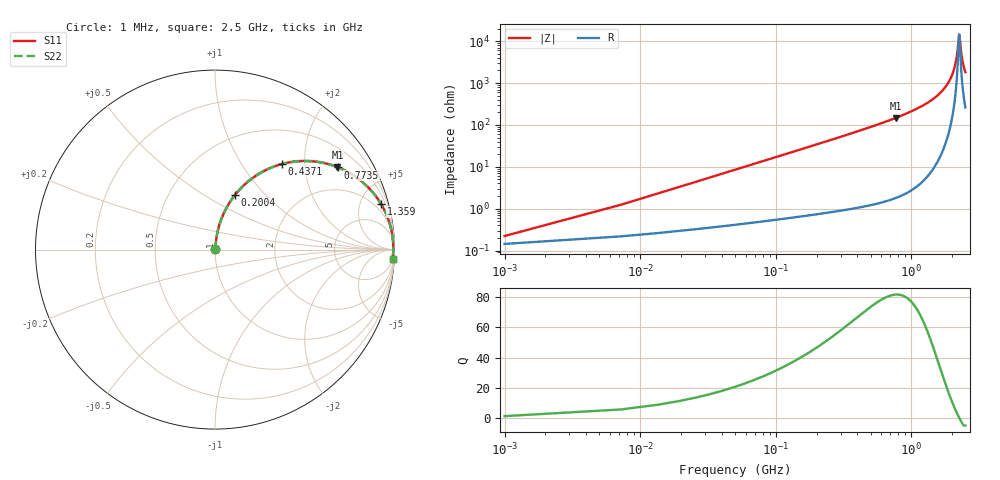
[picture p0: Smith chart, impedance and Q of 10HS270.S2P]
! Coilcraft 1008HS-270 Chip Inductor
! 02 July 2002
# MHZ S MA R 50
!Freq  MagS11  AngS11  MagS21  AngS21  MagS12  AngS12  MagS22  AngS22
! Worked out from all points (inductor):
!   403 points, 1 MHz to 2.5 GHz, reference 50 ohm
!   read as one part in series: L = 27 nH near 13.46 MHz
!   highest Q = 81.7 at 767.3 MHz (marker M1), where L = 30.5 nH
!   self-resonance near 2.25 GHz
!   S11 on the Smith chart (normalised r, x): 1 MHz: 1.00, +0.00; 200.4 MHz: 1.01, +0.69; 437.1 MHz: 1.02, +1.54; 773.5 MHz: 1.04, +2.98; 1.359 GHz: 1.13, +7.25; 2.5 GHz: 6, -36
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1  0.002223 49.6  0.9986 -0.1  0.9986 -0.1  0.002223 49.6
19.69  0.03342 83.0  0.9965 -1.9  0.9965 -1.9  0.03342 83.0
32.15  0.05439 83.2  0.995 -3.1  0.995 -3.1  0.05439 83.2
50.84  0.08572 82.3  0.9922 -4.9  0.9922 -4.9  0.08572 82.3
106.91  0.178 78.0  0.9786 -10.2  0.9786 -10.2  0.178 78.0
200.36  0.3221 70.0  0.9398 -18.8  0.9398 -18.8  0.3221 70.0
418.41  0.5883 53.1  0.8001 -36.0  0.8001 -36.0  0.5883 53.1
437.1  0.6062 51.9  0.7866 -37.3  0.7866 -37.3  0.6062 51.9
767.29  0.8226 34.0  0.5586 -55.3  0.5586 -55.3  0.8226 34.0
773.52  0.8253 33.7  0.5547 -55.6  0.5547 -55.6  0.8253 33.7
835.82  0.8498 31.1  0.5168 -58.2  0.5168 -58.2  0.8498 31.1
1253.23  0.9466 17.9  0.3074 -71.2  0.3074 -71.2  0.9466 17.9
1359.14  0.9595 15.3  0.2646 -73.6  0.2646 -73.6  0.9595 15.3
1670.64  0.9826 9.0  0.156 -79.1  0.156 -79.1  0.9826 9.0
1919.84  0.9908 4.8  0.08336 -81.3  0.08336 -81.3  0.9908 4.8
2088.05  0.9929 2.3  0.03989 -78.7  0.03989 -78.7  0.9929 2.3
2162.81  0.9932 1.2  0.02208 -71.6  0.02208 -71.6  0.9932 1.2
2250.03  0.9931 0.0  0.00688 -4.5  0.00688 -4.5  0.9931 0.0
2268.72  0.9931 -0.2  0.007883 28.2  0.007883 28.2  0.9931 -0.2
2318.56  0.9928 -0.9  0.01665 63.8  0.01665 63.8  0.9928 -0.9
2362.17  0.9924 -1.4  0.02578 72.1  0.02578 72.1  0.9924 -1.4
2500  0.9906 -3.1  0.05472 78.6  0.05472 78.6  0.9906 -3.1
